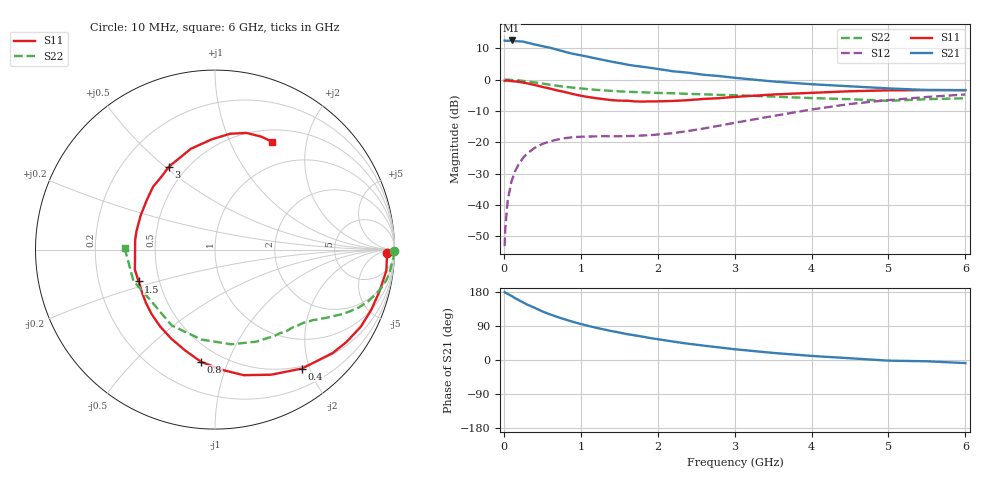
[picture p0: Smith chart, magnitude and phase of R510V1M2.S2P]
! SIEMENS Small Signal Semiconductors
! BFR183
! Si NPN RF Bipolar Junction Transistor in SOT23
! VCE = 10 V  IC = 1.2 mA
! Common Emitter S-Parameters:  May  1996
# GHz  S  MA  R  50
!  f  S11  S21  S12  S22
! GHz  MAG  ANG  MAG  ANG  MAG  ANG  MAG  ANG
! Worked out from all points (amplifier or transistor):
!   36 points, 10 MHz to 6 GHz, reference 50 ohm
!   highest |S21| = 12.5 dB at 100 MHz (marker M1)
!   |S21| within 3 dB of that: start of sweep to 703.3 MHz
!   unconditionally stable (mu >= 1): 1.628 GHz to 2.94 GHz
!   at 250 MHz: K = 0.17, MSG = 18.6 dB, |S12| = -25.0 dB
!   at 1.4 GHz: K = 0.89, MSG = 11.9 dB, |S12| = -18.1 dB
!   at 6 GHz: K = 0.92, MSG = 0.7 dB, |S12| = -4.8 dB
!   S11 on the Smith chart (normalised r, x): 10 MHz: 38, -19; 400 MHz: 0.46, -1.88; 800 MHz: 0.39, -0.81; 1.5 GHz: 0.38, -0.17; 3 GHz: 0.40, +0.52; 6 GHz: 0.65, +1.46
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0.01  0.9587 -1.2  4.2 179.2  0.0022 89.7  0.9969 -0.5
0.02  0.9589 -2.9  4.162 177.6  0.0044 84.4  0.9954 -1.1
0.05  0.9619 -7.0  4.158 174.5  0.0118 85.5  0.9954 -2.6
0.1  0.9453 -14.3  4.207 169.0  0.0239 81.3  0.9867 -5.2
0.15  0.9329 -21.1  4.085 162.8  0.0352 77.5  0.98 -7.9
0.25  0.8954 -35.1  4.04 151.9  0.0563 69.5  0.9523 -12.7
0.3  0.873 -41.3  3.889 146.7  0.0655 66.0  0.9352 -14.9
0.4  0.821 -53.8  3.637 137.9  0.0812 59.4  0.9011 -18.6
0.5  0.7646 -65.7  3.413 128.2  0.0938 53.7  0.8638 -21.9
0.6  0.7179 -77.1  3.221 120.4  0.1036 49.1  0.8259 -24.6
0.8  0.6304 -97.0  2.76 106.8  0.1164 41.7  0.7657 -28.7
0.9  0.5868 -106.3  2.573 100.6  0.1207 39.3  0.7439 -30.3
1.1  0.5265 -125.4  2.302 89.9  0.1236 36.3  0.703 -33.3
1.3  0.4865 -142.2  2.047 80.7  0.125 35.3  0.6719 -35.8
1.5  0.4611 -157.4  1.837 72.6  0.1246 35.9  0.6487 -38.4
1.9  0.4482 173.0  1.541 58.1  0.1297 41.4  0.6203 -43.9
2.2  0.4558 155.4  1.355 48.7  0.1397 46.9  0.6048 -48.5
3  0.5286 119.1  1.067 28.4  0.2042 56.3  0.5632 -65.5
3.5  0.5777 103.4  0.933 18.7  0.2621 55.1  0.5351 -80.3
4.5  0.6509 82.6  0.781 4.6  0.4085 43.7  0.4866 -119.7
5.5  0.6801 67.7  0.682 -3.4  0.5286 27.6  0.4868 -159.0
6  0.6801 62.0  0.676 -8.1  0.578 17.8  0.5037 178.9
